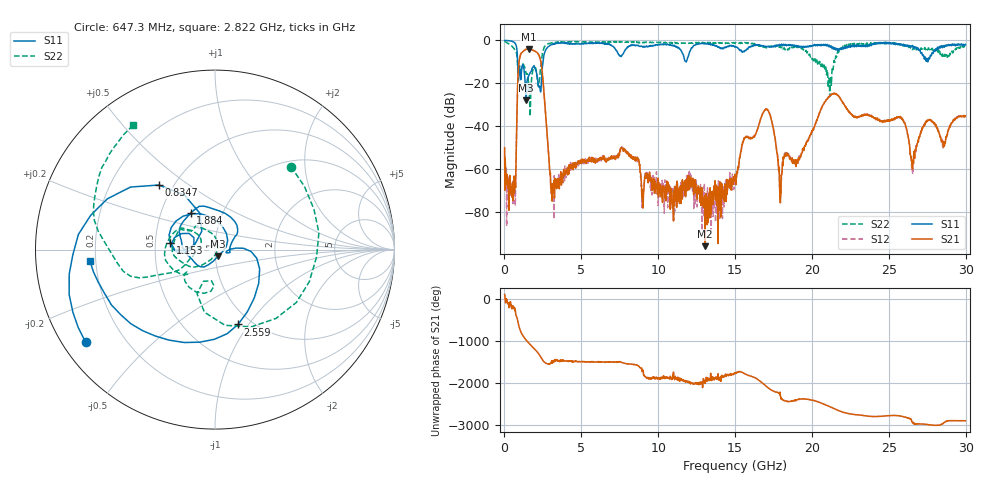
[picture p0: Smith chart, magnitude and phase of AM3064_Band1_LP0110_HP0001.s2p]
# Hz S DB R 50.0
!freq dBS11 angS11 dBS21 angS21 dBS12 angS12 dBS22 angS22
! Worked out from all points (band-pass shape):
!   1600 points, 10 MHz to 29.98 GHz, reference 50 ohm
!   highest |S21| = -4.00 dB at 1.584 GHz (marker M1); lowest = -96.0 dB at 13.06 GHz (marker M2)
!   |S21| within 3 dB of the highest: 1.034 GHz to 2.245 GHz (1.212 GHz wide, 73.9 % of centre)
!   lowest |S11| = -27.9 dB at 1.416 GHz (marker M3), VSWR 1.08, Z = 51.5 - j3.83 ohm
!   |S11| at or under -10 dB: 857.4 MHz to 2.507 GHz (1.65 GHz wide, 98.1 % of centre); 11.80627 GHz to 11.82703 GHz (20.76 MHz wide, 0.176 % of centre)
!   |S22| runs from -35.4 to -0.4 dB; largest |S21 - S12| = 0.011
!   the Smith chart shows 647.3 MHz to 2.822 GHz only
!   S11 on the Smith chart (normalised r, x): 647.3 MHz: 0.07, -0.32; 834.7 MHz: 0.42, +0.39; 1.153 GHz: 0.60, +0.05; 1.884 GHz: 0.71, +0.31; 2.559 GHz: 0.87, -0.89; 2.822 GHz: 0.18, -0.04
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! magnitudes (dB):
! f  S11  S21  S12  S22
! 10 MHz  -0.1  -50.1  -52.9  -0.4
! 647.3 MHz  -1.0  -71.3  -70.0  -4.1
! 834.7 MHz  -6.4  -27.4  -27.4  -9.0
! 1.153 GHz  -11.9  -5.5  -5.5  -11.8
! 1.416 GHz  -27.9  -4.1  -4.1  -15.6
! 1.584 GHz  -16.3  -4.0  -4.0  -20.7
! 1.884 GHz  -12.2  -4.7  -4.8  -12.7
! 2.559 GHz  -7.2  -23.4  -23.3  -3.6
! 2.822 GHz  -3.1  -48.1  -48.1  -1.6
! 3.159 GHz  -1.7  -66.7  -66.7  -1.2
! 5.015 GHz  -1.4  -57.4  -57.0  -0.6
! 7.714 GHz  -6.4  -50.5  -50.9  -0.8
! 10 GHz  -2.0  -64.3  -77.1  -1.0
! 13.06 GHz  -1.6  -96.0  -73.2  -1.3
! 15 GHz  -2.9  -63.1  -64.9  -1.3
! 16.97 GHz  -2.8  -32.3  -32.4  -3.1
! 17.97 GHz  -2.4  -70.4  -73.3  -3.1
! 19.99 GHz  -2.8  -42.4  -42.8  -8.3
! 21.43 GHz  -4.2  -24.7  -24.7  -9.5
! 25 GHz  -1.0  -37.6  -37.2  -1.3
! 26.55 GHz  -2.4  -59.8  -62.4  -4.3
! 29.98 GHz  -1.9  -35.2  -35.4  -3.0
